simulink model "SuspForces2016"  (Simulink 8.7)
settings: Solver=VariableStepAuto  SolverMode=SingleTasking  StartTime=0.0  StopTime=10.0  RelTol=1e-3

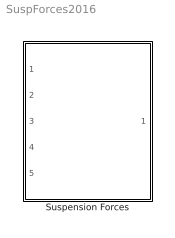
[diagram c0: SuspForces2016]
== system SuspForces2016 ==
  Suspension Forces : Subsystem

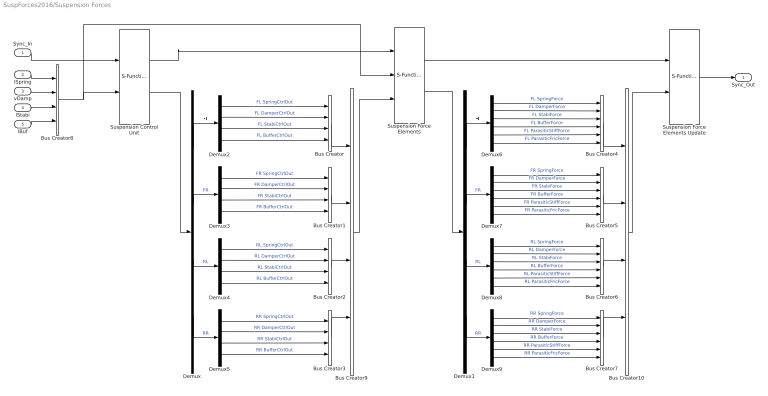
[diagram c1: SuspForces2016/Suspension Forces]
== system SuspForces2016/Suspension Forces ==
  Sync_In : Inport
  lSpring : Inport  Port=2
  vDamp : Inport  Port=3
  lStabi : Inport  Port=4
  lBuf : Inport  Port=5
  Bus Creator{,1..3,8..10} (7 alike) : BusCreator  Inputs=4
  Bus Creator{4..7} (4 alike) : BusCreator  Inputs=6
  Demux{,1..5} (6 alike) : Demux
  Demux{6..9} (4 alike) : Demux  Outputs=6
  Suspension Control Unit : S-Function  FunctionName=CM_Sfun  Parameters='ForcesSuspControl'  SFunctionDeploymentMode=off  EnableBusSupport=off
  Suspension Force Elements : S-Function  FunctionName=CM_Sfun  Parameters='ForcesSusp'  SFunctionDeploymentMode=off  EnableBusSupport=off
  Suspension Force Elements Update : S-Function  FunctionName=CM_Sfun  Parameters='ForcesSuspUpd'  SFunctionDeploymentMode=off  EnableBusSupport=off
  Sync_Out : Outport
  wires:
  vDamp/1 -> Bus Creator8/2
  lStabi/1 -> Bus Creator8/3
  lBuf/1 -> Bus Creator8/4
  lSpring/1 -> Bus Creator8/1
  Bus Creator8/1 -> Suspension Control Unit/2, Suspension Force Elements/2
  Sync_In/1 -> Suspension Control Unit/1
  Suspension Control Unit/1 -> Suspension Force Elements/1
  Suspension Force Elements/1 -> Suspension Force Elements Update/1
  Suspension Force Elements Update/1 -> Sync_Out/1
  Bus Creator4/1 -> Bus Creator10/1
  Bus Creator5/1 -> Bus Creator10/2
  Bus Creator6/1 -> Bus Creator10/3
  Bus Creator7/1 -> Bus Creator10/4
  Demux6/1 -> Bus Creator4/1  "FL SpringForce"
  Demux9/1 -> Bus Creator7/1  "RR SpringForce"
  Demux9/2 -> Bus Creator7/2  "RR DamperForce"
  Demux9/3 -> Bus Creator7/3  "RR StabiForce"
  Demux9/4 -> Bus Creator7/4  "RR BufferForce"
  Demux9/5 -> Bus Creator7/5  "RR ParasiticStiffForce"
  Demux9/6 -> Bus Creator7/6  "RR ParasiticFricForce"
  Demux8/1 -> Bus Creator6/1  "RL SpringForce"
  Demux8/2 -> Bus Creator6/2  "RL DamperForce"
  Demux8/4 -> Bus Creator6/4  "RL BufferForce"
  Demux8/5 -> Bus Creator6/5  "RL ParasiticStiffForce"
  Demux8/6 -> Bus Creator6/6  "RL ParasiticFricForce"
  Demux8/3 -> Bus Creator6/3  "RL StabiForce"
  Demux7/1 -> Bus Creator5/1  "FR SpringForce"
  Demux7/2 -> Bus Creator5/2  "FR DamperForce"
  Demux7/3 -> Bus Creator5/3  "FR StabiForce"
  Demux7/4 -> Bus Creator5/4  "FR BufferForce"
  Demux7/5 -> Bus Creator5/5  "FR ParasiticStiffForce"
  Demux7/6 -> Bus Creator5/6  "FR ParasiticFricForce"
  Demux6/2 -> Bus Creator4/2  "FL DamperForce"
  Demux6/3 -> Bus Creator4/3  "FL StabiForce"
  Demux6/4 -> Bus Creator4/4  "FL BufferForce"
  Demux6/5 -> Bus Creator4/5  "FL ParasiticStiffForce"
  Demux6/6 -> Bus Creator4/6  "FL ParasiticFricForce"
  Bus Creator10/1 -> Suspension Force Elements Update/2
  Demux/1 -> Demux2/1  "FL"
  Bus Creator1/1 -> Bus Creator9/2
  Demux/2 -> Demux3/1  "FR"
  Bus Creator2/1 -> Bus Creator9/3
  Demux/3 -> Demux4/1  "RL"
  Bus Creator3/1 -> Bus Creator9/4
  Demux2/1 -> Bus Creator/1  "FL SpringCtrlOut"
  Demux/4 -> Demux5/1  "RR"
  Demux5/1 -> Bus Creator3/1  "RR SpringCtrlOut"
  Demux5/2 -> Bus Creator3/2  "RR DamperCtrlOut"
  Demux5/3 -> Bus Creator3/3  "RR StabiCtrlOut"
  Demux5/4 -> Bus Creator3/4  "RR BufferCtrlOut"
  Demux4/1 -> Bus Creator2/1  "RL SpringCtrlOut"
  Demux4/2 -> Bus Creator2/2  "RL DamperCtrlOut"
  Demux4/4 -> Bus Creator2/4  "RL BufferCtrlOut"
  Demux4/3 -> Bus Creator2/3  "RL StabiCtrlOut"
  Demux3/1 -> Bus Creator1/1  "FR SpringCtrlOut"
  Demux3/2 -> Bus Creator1/2  "FR DamperCtrlOut"
  Demux3/3 -> Bus Creator1/3  "FR StabiCtrlOut"
  Demux3/4 -> Bus Creator1/4  "FR BufferCtrlOut"
  Demux2/2 -> Bus Creator/2  "FL DamperCtrlOut"
  Demux2/3 -> Bus Creator/3  "FL StabiCtrlOut"
  Demux2/4 -> Bus Creator/4  "FL BufferCtrlOut"
  Suspension Control Unit/2 -> Demux/1
  Bus Creator9/1 -> Suspension Force Elements/3
  Bus Creator/1 -> Bus Creator9/1
  Suspension Force Elements/2 -> Demux1/1
  Demux1/1 -> Demux6/1  "FL"
  Demux1/2 -> Demux7/1  "FR"
  Demux1/3 -> Demux8/1  "RL"
  Demux1/4 -> Demux9/1  "RR"
